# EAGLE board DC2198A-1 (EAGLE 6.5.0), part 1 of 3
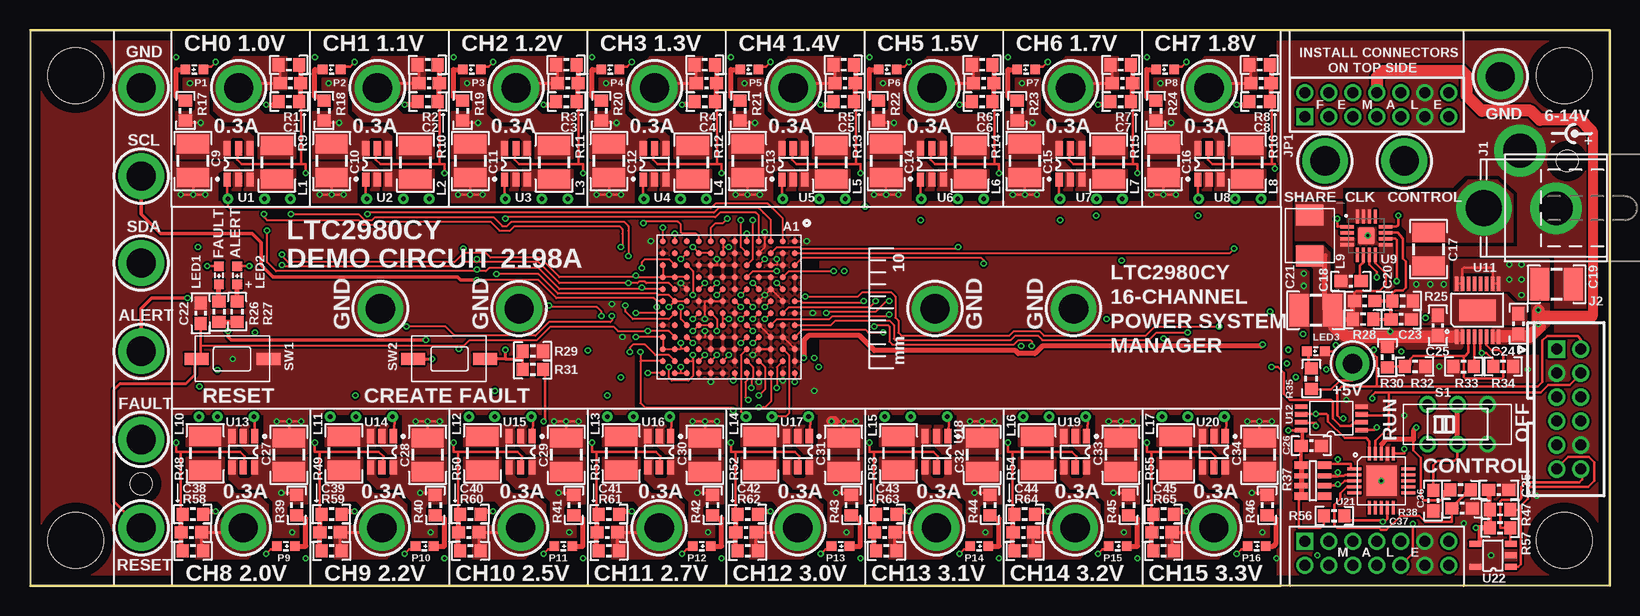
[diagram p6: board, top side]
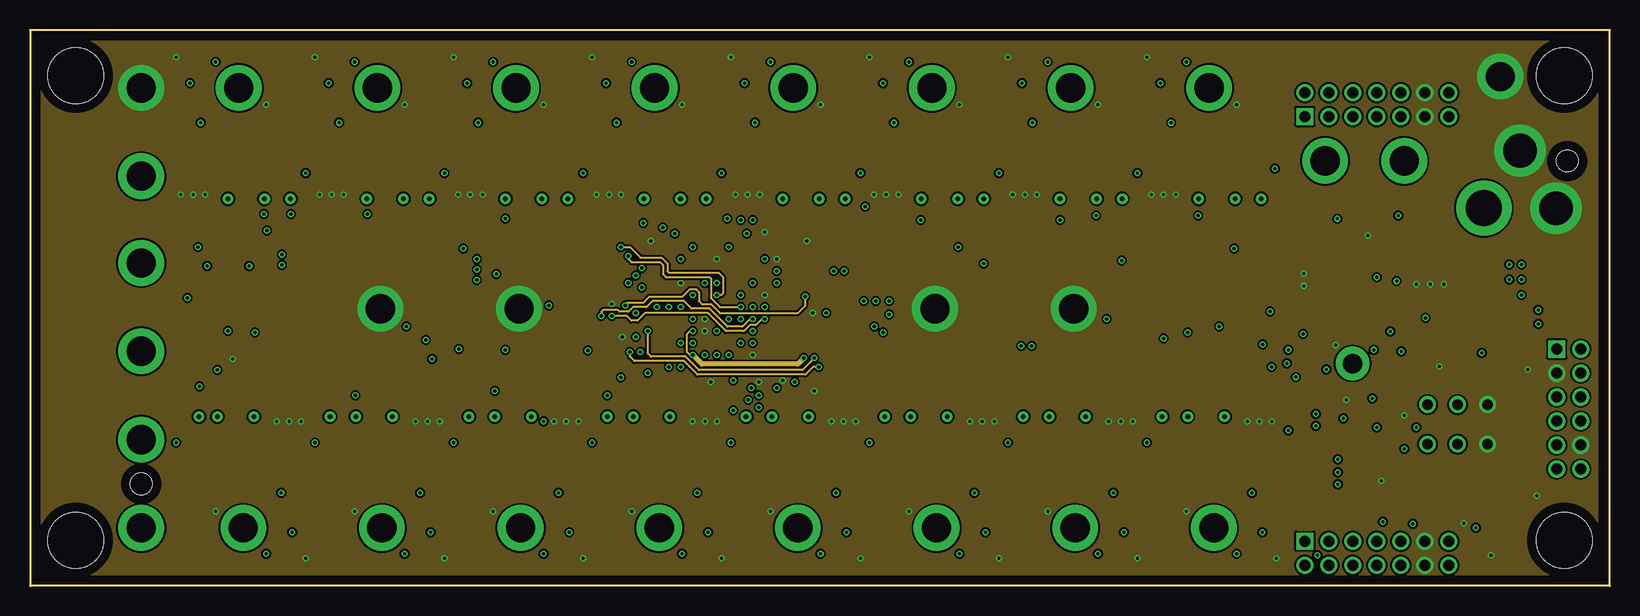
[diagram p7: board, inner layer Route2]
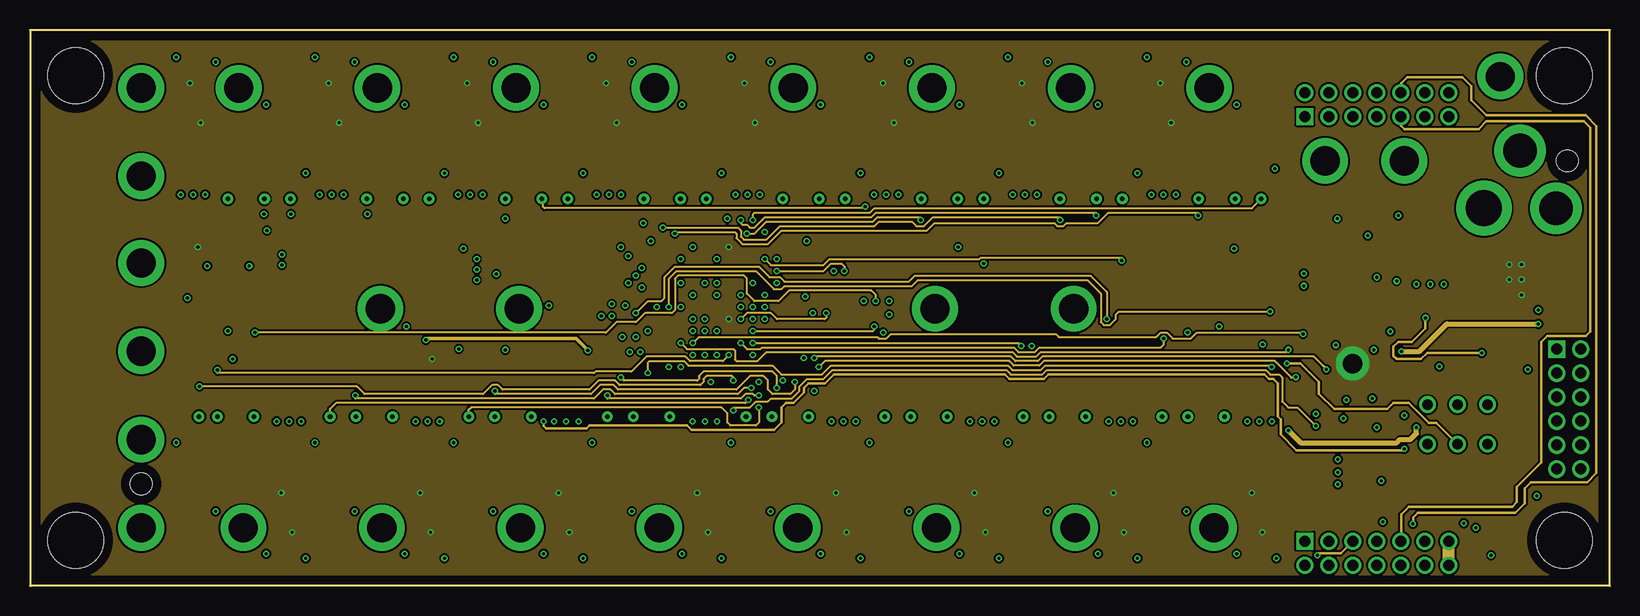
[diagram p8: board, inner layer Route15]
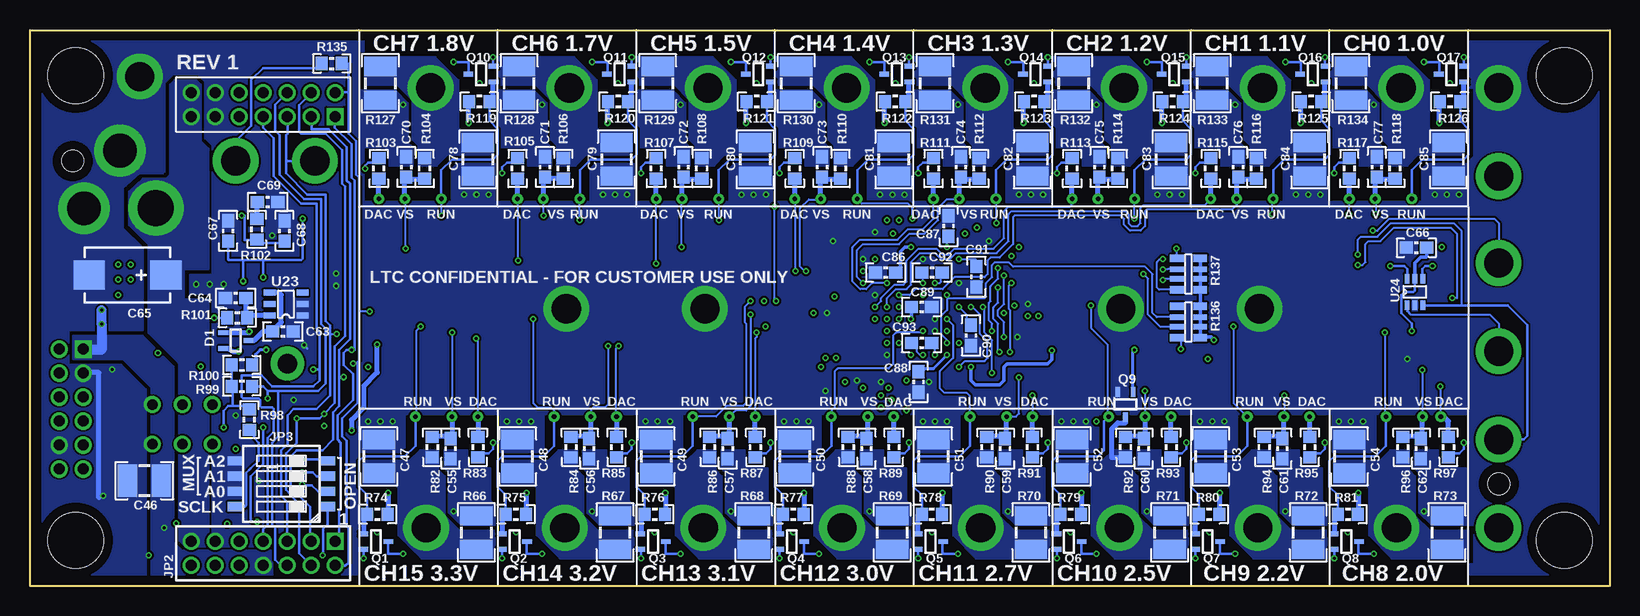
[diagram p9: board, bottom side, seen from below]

Size 131.7 x 46.35 mm. Coordinates in mm from the lower left corner, seen from the top.
Outline: 0,0 0,46.35 131.7,46.35 131.7,0 0.13,0
Copper layers (1*2+15*16): Top 0.035mm / dielectric 1.5mm / Route2 0.035mm / dielectric 0.15mm / Route15 0.035mm / dielectric 0.2mm / Bottom 0.035mm
Design rules "default *": minimum track width 6.5mil, minimum drill 10mil, track to track 0.16mm, track to pad 0.16mm, pad to pad 0.16mm, via to via 0.16mm, smd to smd 0.05mm, copper to edge 30mil, drill to drill 20mil, minimum pad ring 10mil, minimum via ring 5mil, stop-mask expansion 4mil, vias tented up to drill 16mil, thermal gap 10mil
Holes 4.65 mm at 3.81,3.81 3.81,42.55 127.89,42.55 127.89,3.81
Holes 1.8 mm at 9.27,8.51 128.14,35.43

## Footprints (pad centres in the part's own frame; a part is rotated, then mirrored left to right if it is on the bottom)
C0603_BOX = smd 1.1 x 1: 1 -0.85,0; 2 0.85,0
C1210_BOX = smd 1.6 x 2.7: 1 -1.4,0; 2 1.4,0
C7343 = smd 2.6 x 2.4: + -3.2,0; - 3.2,0
SC70-3 = smd 0.4 x 0.8: 1 -0.65,-1.052; 2 0.65,-1.052; 3 0,1.052
PJ-002A = drill 3 pad 4.6: 1 3,0 | drill 2.8 pad 4.3: 2 -3,0; 3 0,-4.8
CONN_DC1613 = drill 0.914 square: 1 -5,-1 | drill 0.914: 2 -5,1; 3 -3,-1; 4 -3,1; 5 -1,-1; 6 -1,1; 7 1,-1; 8 1,1; 9 3,-1; 10 3,1; 11 5,-1; 12 5,1
2X07M = drill 0.914 square: 1 -6,-1 | drill 0.914: 2 -6,1; 3 -4,-1; 4 -4,1; 5 -2,-1; 6 -2,1; 7 0,-1; 8 0,1; 9 2,-1; 10 2,1; 11 4,-1; 12 4,1; 13 6,-1; 14 6,1
SMT_DIP_4 = smd 1.27 x 0.762: 1 -3.861,1.905; 2 -3.861,0.635; 3 -3.861,-0.635; 4 -3.861,-1.905; 5 3.861,-1.905; 6 3.861,-0.635; 7 3.861,0.635; 8 3.861,1.905
L1210 = smd 1.6 x 2.7: 1 -1.4,0; 2 1.4,0
IHLP_1616AB = smd 1.75 x 2.3: 1 -1.7,0; 2 1.7,0
CHIPLED_0603 = smd 0.8 x 0.8: N 0,0.75; P 0,-0.75
R0603_BOX = smd 1 x 1.1: 1 -0.85,0; 2 0.85,0
R_VISHAY_CRA06S = smd 1.15 x 0.63: R1_1 -0.975,1.295; R1_2 0.975,1.295; R4_1 -0.975,-1.295; R4_2 0.975,-1.295 | smd 1.15 x 0.44: R2_1 -0.975,0.4; R2_2 0.975,0.4; R3_1 -0.975,-0.4; R3_2 0.975,-0.4
R1210_BOX = smd 1.6 x 2.7: 1 -1.4,0; 2 1.4,0
JS202011CQN = drill 0.9: 1 -2.5,1.65; 2 0,1.65; 3 2.5,1.65; 4 -2.5,-1.65; 5 0,-1.65; 6 2.5,-1.65
SWITCH_PTS635 = smd 2 x 1: SW1 -3,0; SW2 3,0
TP1 = drill 2.438 pad 3.81: TP 0,0
TURRET_SMALL_2308 = drill 1.626 pad 2.794: TP1 0,0
SOT-23-6 = smd 1.2 x 0.6: 1 -1.3,0.95; 2 -1.3,0; 3 -1.3,-0.95; 4 1.3,-0.95; 5 1.3,0; 6 1.3,0.95
QFN16_3X3 = smd 1.2 x 0.3: 1 -1.711,0.734; 2 -1.711,0.234; 3 -1.711,-0.266; 4 -1.711,-0.766; 9 1.489,-0.766; 10 1.489,-0.266; 11 1.489,0.234; 12 1.489,0.734 | smd 0.3 x 1.2: 5 -0.861,-1.616; 6 -0.361,-1.616; 7 0.139,-1.616; 8 0.639,-1.616; 13 0.639,1.584; 14 0.139,1.584; 15 -0.361,1.584; 16 -0.861,1.584 | smd 1.4 x 1.4: PAD -0.111,-0.016
BGA_144_1.0 = smd 0.5 x 0.5: A1 -5.5,5.5; A2 -4.5,5.5; A3 -3.5,5.5; A4 -2.5,5.5; A5 -1.5,5.5; A6 -0.5,5.5; A7 0.5,5.5; A8 1.5,5.5; A9 2.5,5.5; A10 3.5,5.5; A11 4.5,5.5; A12 5.5,5.5; B1 -5.5,4.5; B2 -4.5,4.5; B3 -3.5,4.5; B4 -2.5,4.5; B5 -1.5,4.5; B6 -0.5,4.5; B7 0.5,4.5; B8 1.5,4.5; B9 2.5,4.5; B10 3.5,4.5; B11 4.5,4.5; B12 5.5,4.5; C1 -5.5,3.5; C2 -4.5,3.5; C3 -3.5,3.5; C4 -2.5,3.5; C5 -1.5,3.5; C6 -0.5,3.5; C7 0.5,3.5; C8 1.5,3.5; C9 2.5,3.5; C10 3.5,3.5; C11 4.5,3.5; C12 5.5,3.5; D1 -5.5,2.5; D2 -4.5,2.5; D3 -3.5,2.5; D4 -2.5,2.5; D5 -1.5,2.5; D6 -0.5,2.5; D7 0.5,2.5; D8 1.5,2.5; D9 2.5,2.5; D10 3.5,2.5; D11 4.5,2.5; D12 5.5,2.5; E1 -5.5,1.5; E2 -4.5,1.5; E3 -3.5,1.5; E4 -2.5,1.5; E5 -1.5,1.5; E6 -0.5,1.5; E7 0.5,1.5; E8 1.5,1.5; E9 2.5,1.5; E10 3.5,1.5; E11 4.5,1.5; E12 5.5,1.5; F1 -5.5,0.5; F2 -4.5,0.5; F3 -3.5,0.5; F4 -2.5,0.5; F5 -1.5,0.5; F6 -0.5,0.5; F7 0.5,0.5; F8 1.5,0.5; F9 2.5,0.5; F10 3.5,0.5; F11 4.5,0.5; F12 5.5,0.5; G1 -5.5,-0.5; G2 -4.5,-0.5; G3 -3.5,-0.5; G4 -2.5,-0.5; G5 -1.5,-0.5; G6 -0.5,-0.5; G7 0.5,-0.5; G8 1.5,-0.5; G9 2.5,-0.5; G10 3.5,-0.5; G11 4.5,-0.5; G12 5.5,-0.5; H1 -5.5,-1.5; H2 -4.5,-1.5; H3 -3.5,-1.5; H4 -2.5,-1.5; H5 -1.5,-1.5; H6 -0.5,-1.5; H7 0.5,-1.5; H8 1.5,-1.5; H9 2.5,-1.5; H10 3.5,-1.5; H11 4.5,-1.5; H12 5.5,-1.5; J1 -5.5,-2.5; J2 -4.5,-2.5; J3 -3.5,-2.5; J4 -2.5,-2.5; J5 -1.5,-2.5; J6 -0.5,-2.5; J7 0.5,-2.5; J8 1.5,-2.5; J9 2.5,-2.5; J10 3.5,-2.5; J11 4.5,-2.5; J12 5.5,-2.5; K1 -5.5,-3.5; K2 -4.5,-3.5; K3 -3.5,-3.5; K4 -2.5,-3.5; K5 -1.5,-3.5; K6 -0.5,-3.5; K7 0.5,-3.5; K8 1.5,-3.5; K9 2.5,-3.5; K10 3.5,-3.5; K11 4.5,-3.5; K12 5.5,-3.5; L1 -5.5,-4.5; L2 -4.5,-4.5; L3 -3.5,-4.5; L4 -2.5,-4.5; L5 -1.5,-4.5; L6 -0.5,-4.5; L7 0.5,-4.5; L8 1.5,-4.5; L9 2.5,-4.5; L10 3.5,-4.5; L11 4.5,-4.5; L12 5.5,-4.5; M1 -5.5,-5.5; M2 -4.5,-5.5; M3 -3.5,-5.5; M4 -2.5,-5.5; M5 -1.5,-5.5; M6 -0.5,-5.5; M7 0.5,-5.5; M8 1.5,-5.5; M9 2.5,-5.5; M10 3.5,-5.5; M11 4.5,-5.5; M12 5.5,-5.5
MSOP16_EXP = smd 1.2 x 0.3: 1 -2.213,1.75; 2 -2.213,1.25; 3 -2.213,0.75; 4 -2.213,0.25; 5 -2.213,-0.25; 6 -2.213,-0.75; 7 -2.213,-1.25; 8 -2.213,-1.75; 9 2.213,-1.75; 10 2.213,-1.25; 11 2.213,-0.75; 12 2.213,-0.25; 13 2.213,0.25; 14 2.213,0.75; 15 2.213,1.25; 16 2.213,1.75 | smd 1.778 x 3.048: EXP 0,0
MSOP-8 = smd 1.041 x 0.381: 1 -2.55,0.975; 2 -2.55,0.325; 3 -2.55,-0.325; 4 -2.55,-0.975; 5 2.479,-0.975; 6 2.479,-0.325; 7 2.479,0.325; 8 2.479,0.975
QFN20 = smd 1.143 x 0.254: 1 -2.25,1; 2 -2.25,0.5; 3 -2.25,0; 4 -2.25,-0.5; 5 -2.25,-1; 11 2.25,-1; 12 2.25,-0.5; 13 2.25,0; 14 2.25,0.5; 15 2.25,1 | smd 0.254 x 1.143: 6 -1,-2.25; 7 -0.5,-2.25; 8 0,-2.25; 9 0.5,-2.25; 10 1,-2.25; 16 1,2.25; 17 0.5,2.25; 18 0,2.25; 19 -0.5,2.25; 20 -1,2.25 | smd 2.54 x 2.54: PAD 0,0
SOT-23-5 = smd 1 x 0.5: 1 -1.649,0.95; 2 -1.649,0; 3 -1.649,-0.95; 4 1.333,-0.95; 5 1.333,0.95
SOT-23-6@1 = smd 1 x 0.5: 1 -1.374,1.087; 2 -1.374,0.127; 3 -1.374,-0.833; 4 1.374,-0.833; 5 1.374,0.127; 6 1.374,1.087
SC70-6 = smd 0.4 x 0.8: 1 -0.65,-1.102; 2 0,-1.102; 3 0.65,-1.102; 4 0.65,1.102; 5 0,1.098; 6 -0.65,1.102
VIA = drill 0.381: 1 0,0

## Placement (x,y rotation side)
$$U$1  [LT_LOGO_LARGE_SM]  5.46,6.1 90 top
$$U$2  [LT_LOGO_LARGE_SM]  2.03,6.1 90 bottom
C1  220p  [C0603_BOX]  21.72,41.91 0 top
C2  220p  [C0603_BOX]  33.27,41.91 0 top
C3  220p  [C0603_BOX]  44.83,41.91 0 top
C4  220p  [C0603_BOX]  56.39,41.91 0 top
C5  220p  [C0603_BOX]  67.94,41.91 0 top
C6  220p  [C0603_BOX]  79.5,41.91 0 top
C7  220p  [C0603_BOX]  91.06,41.91 0 top
C8  220p  [C0603_BOX]  102.62,41.91 0 top
C9  10u/10V  [C1210_BOX]  13.59,35.43 270 top
C10  10u/10V  [C1210_BOX]  25.15,35.43 270 top
C11  10u/10V  [C1210_BOX]  36.7,35.43 270 top
C12  10u/10V  [C1210_BOX]  48.26,35.43 270 top
C13  10u/10V  [C1210_BOX]  59.82,35.43 270 top
C14  10u/10V  [C1210_BOX]  71.37,35.43 270 top
C15  10u/10V  [C1210_BOX]  82.93,35.43 270 top
C16  10u/10V  [C1210_BOX]  94.49,35.43 270 top
C17  10u/25V  [C1210_BOX]  116.59,28.07 90 top
C18  100n  [C0603_BOX]  110.11,25.4 0 top
C19  10u/10V  [C1210_BOX]  127.25,25.15 0 top
C20  68p  [C0603_BOX]  111.25,23.75 0 top
C21  22u/10V  [C1210_BOX]  107.19,22.99 180 top
C22  10n  [C0603_BOX]  14.22,22.73 90 top
C23  47p  [C0603_BOX]  114.3,22.23 0 top
C24  1u  [C0603_BOX]  124.08,21.84 90 top
C25  1u  [C0603_BOX]  117.35,21.72 90 top
C26  100n  [C0603_BOX]  106.81,11.68 0 top
C27  10u/10V  [C1210_BOX]  21.59,10.92 90 top
C28  10u/10V  [C1210_BOX]  33.15,10.92 90 top
C29  10u/10V  [C1210_BOX]  44.7,10.92 90 top
C30  10u/10V  [C1210_BOX]  56.26,10.92 90 top
C31  10u/10V  [C1210_BOX]  67.82,10.92 90 top
C32  10u/10V  [C1210_BOX]  79.38,10.92 90 top
C33  10u/10V  [C1210_BOX]  90.93,10.92 90 top
C34  10u/10V  [C1210_BOX]  102.49,10.92 90 top
C35  1u  [C0603_BOX]  122.43,8 0 top
C36  1u  [C0603_BOX]  116.97,7.11 270 top
C37  1u  [C0603_BOX]  119.38,6.48 0 top
C38  220p  [C0603_BOX]  13.46,4.45 180 top
C39  220p  [C0603_BOX]  25.02,4.45 180 top
C40  220p  [C0603_BOX]  36.58,4.45 180 top
C41  220p  [C0603_BOX]  48.13,4.45 180 top
C42  220p  [C0603_BOX]  59.69,4.45 180 top
C43  220p  [C0603_BOX]  71.25,4.45 180 top
C44  220p  [C0603_BOX]  82.8,4.45 180 top
C45  220p  [C0603_BOX]  94.36,4.45 180 top
C46  10u/10V  [C1210_BOX]  122.17,8.76 180 bottom
C47  22u/10V  [C1210_BOX]  102.62,10.79 90 bottom
C48  22u/10V  [C1210_BOX]  91.06,10.79 90 bottom
C49  22u/10V  [C1210_BOX]  79.5,10.79 90 bottom
C50  22u/10V  [C1210_BOX]  67.94,10.79 90 bottom
C51  22u/10V  [C1210_BOX]  56.39,10.79 90 bottom
C52  22u/10V  [C1210_BOX]  44.83,10.79 90 bottom
C53  22u/10V  [C1210_BOX]  33.27,10.79 90 bottom
C54  22u/10V  [C1210_BOX]  21.72,10.79 90 bottom
C55  100n  [C0603_BOX]  96.65,11.43 90 bottom
C56  100n  [C0603_BOX]  85.09,11.43 90 bottom
C57  100n  [C0603_BOX]  73.53,11.43 90 bottom
C58  100n  [C0603_BOX]  61.98,11.43 90 bottom
C59  100n  [C0603_BOX]  50.42,11.43 90 bottom
C60  100n  [C0603_BOX]  38.86,11.43 90 bottom
C61  100n  [C0603_BOX]  27.3,11.43 90 bottom
C62  100n  [C0603_BOX]  15.75,11.43 90 bottom
C63  1u  [C0603_BOX]  110.62,21.21 0 bottom
C64  4.7u  [C0603_BOX]  114.55,24 0 bottom
C65  47u/16V  [C7343]  123.57,25.91 180 bottom
C66  1u  [C0603_BOX]  16.13,28.19 180 bottom
C67  4.7u  [C0603_BOX]  115.19,29.59 90 bottom
C68  4.7p  [C0603_BOX]  110.49,29.59 90 bottom
C69  68p  [C0603_BOX]  111.89,32 0 bottom
C70  100n  [C0603_BOX]  100.33,34.92 270 bottom
C71  100n  [C0603_BOX]  88.77,34.92 270 bottom
C72  100n  [C0603_BOX]  77.22,34.92 270 bottom
C73  100n  [C0603_BOX]  65.66,34.92 270 bottom
C74  100n  [C0603_BOX]  54.1,34.92 270 bottom
C75  100n  [C0603_BOX]  42.55,34.92 270 bottom
C76  100n  [C0603_BOX]  30.99,34.92 270 bottom
C77  100n  [C0603_BOX]  19.43,34.92 270 bottom
C78  22u/10V  [C1210_BOX]  94.36,35.56 270 bottom
C79  22u/10V  [C1210_BOX]  82.8,35.56 270 bottom
C80  22u/10V  [C1210_BOX]  71.25,35.56 270 bottom
C81  22u/10V  [C1210_BOX]  59.69,35.56 270 bottom
C82  22u/10V  [C1210_BOX]  48.13,35.56 270 bottom
C83  22u/10V  [C1210_BOX]  36.58,35.56 270 bottom
C84  22u/10V  [C1210_BOX]  25.02,35.56 270 bottom
C85  22u/10V  [C1210_BOX]  13.46,35.56 270 bottom
C86  100n  [C0603_BOX]  60.38,26.12 180 bottom
C87  100n  [C0603_BOX]  55.12,30 90 bottom
C88  100n  [C0603_BOX]  57.62,17 90 bottom
C89  100n  [C0603_BOX]  57.38,23.25 0 bottom
C90  100n  [C0603_BOX]  53.25,20.88 90 bottom
C91  100n  [C0603_BOX]  52.81,25.78 90 bottom
C92  100n  [C0603_BOX]  56.5,26.12 180 bottom
C93  100n  [C0603_BOX]  57.38,20.25 180 bottom
D1  BAT30CWFILM  [SC70-3]  114.55,20.45 270 bottom
DRILEGEND  [DRILEGEND]  not placed on the board
J1  PJ-002A  [PJ-002A]  124.21,31.5 180 top
J2  CONN_DC1613  [CONN_DC1613]  128.27,14.73 270 top
JP1  FEMALE  [2X07M]  112.27,40.13 0 top
JP2  MALE  [2X07M]  112.27,2.72 180 bottom
JP3  TDA04H0SK1  [SMT_DIP_4]  110.74,8.51 0 bottom
L1  4.7uH  [L1210]  20.57,35.31 90 top
L2  4.7uH  [L1210]  32.13,35.31 90 top
L3  4.7uH  [L1210]  43.69,35.31 90 top
L4  4.7uH  [L1210]  55.24,35.31 90 top
L5  4.7uH  [L1210]  66.8,35.31 90 top
L6  4.7uH  [L1210]  78.36,35.31 90 top
L7  4.7uH  [L1210]  89.92,35.31 90 top
L8  4.7uH  [L1210]  101.47,35.31 90 top
L9  2.2uH  [IHLP_1616AB]  106.68,29.21 270 top
L10  4.7uH  [L1210]  14.61,11.05 270 top
L11  4.7uH  [L1210]  26.16,11.05 270 top
L12  4.7uH  [L1210]  37.72,11.05 270 top
L13  4.7uH  [L1210]  49.28,11.05 270 top
L14  4.7uH  [L1210]  60.83,11.05 270 top
L15  4.7uH  [L1210]  72.39,11.05 270 top
L16  4.7uH  [L1210]  83.95,11.05 270 top
L17  4.7uH  [L1210]  95.5,11.05 270 top
LED1  RED  [CHIPLED_0603]  15.75,25.91 0 top
LED2  RED  [CHIPLED_0603]  17.27,25.91 0 top
LED3  GREEN  [CHIPLED_0603]  107.19,19.56 270 top
P1  GREEN  [CHIPLED_0603]  13.72,43.05 270 top
P2  GREEN  [CHIPLED_0603]  25.15,43.05 270 top
P3  GREEN  [CHIPLED_0603]  36.83,43.05 270 top
P4  GREEN  [CHIPLED_0603]  48.39,43.05 270 top
P5  GREEN  [CHIPLED_0603]  59.94,43.05 270 top
P6  GREEN  [CHIPLED_0603]  71.5,43.05 270 top
P7  GREEN  [CHIPLED_0603]  83.06,43.05 270 top
P8  GREEN  [CHIPLED_0603]  94.61,43.05 270 top
P9  GREEN  [CHIPLED_0603]  21.34,3.3 90 top
P10  GREEN  [CHIPLED_0603]  32.89,3.3 90 top
P11  GREEN  [CHIPLED_0603]  44.45,3.3 90 top
P12  GREEN  [CHIPLED_0603]  56.01,3.3 90 top
P13  GREEN  [CHIPLED_0603]  67.56,3.3 90 top
P14  GREEN  [CHIPLED_0603]  79.12,3.3 90 top
P15  GREEN  [CHIPLED_0603]  90.68,3.3 90 top
P16  GREEN  [CHIPLED_0603]  102.23,3.3 90 top
Q1  Si1308EDL  [SC70-3]  102.87,3.68 270 bottom
Q2  Si1308EDL  [SC70-3]  91.31,3.68 270 bottom
Q3  Si1308EDL  [SC70-3]  79.76,3.68 270 bottom
Q4  Si1308EDL  [SC70-3]  68.2,3.68 270 bottom
Q5  Si1308EDL  [SC70-3]  56.64,3.68 270 bottom
Q6  Si1308EDL  [SC70-3]  45.09,3.68 270 bottom
Q7  Si1308EDL  [SC70-3]  33.53,3.68 270 bottom
Q8  Si1308EDL  [SC70-3]  21.97,3.68 270 bottom
Q9  Si1308EDL  [SC70-3]  40.39,15.11 180 bottom
Q10  Si1308EDL  [SC70-3]  94.11,42.67 90 bottom
Q11  Si1308EDL  [SC70-3]  82.55,42.67 90 bottom
Q12  Si1308EDL  [SC70-3]  70.99,42.67 90 bottom
Q13  Si1308EDL  [SC70-3]  59.44,42.67 90 bottom
Q14  Si1308EDL  [SC70-3]  47.88,42.67 90 bottom
Q15  Si1308EDL  [SC70-3]  36.32,42.67 90 bottom
Q16  Si1308EDL  [SC70-3]  24.77,42.67 90 bottom
Q17  Si1308EDL  [SC70-3]  13.21,42.67 90 bottom
R1  100k  [R0603_BOX]  21.59,43.43 180 top
R2  100k  [R0603_BOX]  33.15,43.43 180 top
R3  100k  [R0603_BOX]  44.7,43.43 180 top
R4  100k  [R0603_BOX]  56.26,43.43 180 top
R5  100k  [R0603_BOX]  67.82,43.43 180 top
R6  100k  [R0603_BOX]  79.38,43.43 180 top
R7  100k  [R0603_BOX]  90.93,43.43 180 top
R8  100k  [R0603_BOX]  102.49,43.43 180 top
R9  402k  [R0603_BOX]  21.59,40.39 0 top
R10  267k  [R0603_BOX]  33.15,40.39 0 top
R11  200k  [R0603_BOX]  44.7,40.39 0 top
R12  158k  [R0603_BOX]  56.26,40.39 0 top
R13  133k  [R0603_BOX]  67.82,40.39 0 top
R14  115k  [R0603_BOX]  79.38,40.39 0 top
R15  88.7k  [R0603_BOX]  90.93,40.39 0 top
R16  80.6k  [R0603_BOX]  102.49,40.39 0 top
R17  3.01k  [R0603_BOX]  12.95,39.62 270 top
R18  3.01k  [R0603_BOX]  24.51,39.62 270 top
R19  3.01k  [R0603_BOX]  36.07,39.62 270 top
R20  3.01k  [R0603_BOX]  47.62,39.62 270 top
R21  3.01k  [R0603_BOX]  59.18,39.62 270 top
R22  3.01k  [R0603_BOX]  70.74,39.62 270 top
R23  3.01k  [R0603_BOX]  82.3,39.62 270 top
R24  3.01k  [R0603_BOX]  93.85,39.62 270 top
R25  10k  [R0603_BOX]  114.43,23.75 180 top
R26  698  [R0603_BOX]  15.75,22.86 90 top
R27  698  [R0603_BOX]  17.27,22.86 270 top
R28  73.2k  [R0603_BOX]  111.12,22.23 180 top
R29  100k  [R0603_BOX]  41.91,19.56 180 top
R30  46.4k  [R0603_BOX]  113.16,19.05 90 top
R31  OPT  [R0603_BOX]  41.91,18.04 180 top
R32  10k  [R0603_BOX]  115.44,18.29 180 top
R33  249  [R0603_BOX]  119.51,18.29 0 top
R34  1.0k  [R0603_BOX]  122.81,18.29 180 top
R35  3.01k  [R0603_BOX]  106.81,17.27 270 top
R37  10k, 4X  [R_VISHAY_CRA06S]  106.93,8.76 180 top
R38  249  [R0603_BOX]  119.25,8 0 top
R39  3.01k  [R0603_BOX]  22.23,6.73 90 top
R40  3.01k  [R0603_BOX]  33.78,6.73 90 top
R41  3.01k  [R0603_BOX]  45.34,6.73 90 top
R42  3.01k  [R0603_BOX]  56.9,6.73 90 top
R43  3.01k  [R0603_BOX]  68.45,6.73 90 top
R44  3.01k  [R0603_BOX]  80.01,6.73 90 top
R45  3.01k  [R0603_BOX]  91.57,6.73 90 top
R46  3.01k  [R0603_BOX]  103.12,6.73 90 top
R47  10k  [R0603_BOX]  122.56,6.35 180 top
R48  66.5k  [R0603_BOX]  13.59,5.97 180 top
R49  57.6k  [R0603_BOX]  25.15,5.97 180 top
R50  47.5k  [R0603_BOX]  36.7,5.97 180 top
R51  42.2k  [R0603_BOX]  48.26,5.97 180 top
R52  36.5k  [R0603_BOX]  59.82,5.97 180 top
R53  34.8k  [R0603_BOX]  71.37,5.97 180 top
R54  33.2k  [R0603_BOX]  82.93,5.97 180 top
R55  32.4k  [R0603_BOX]  94.49,5.97 180 top
R56  10k  [R0603_BOX]  108.71,5.84 0 top
R57  10k  [R0603_BOX]  122.56,4.83 180 top
R58  100k  [R0603_BOX]  13.59,2.92 0 top
R59  100k  [R0603_BOX]  25.15,2.92 0 top
R60  100k  [R0603_BOX]  36.7,2.92 0 top
R61  100k  [R0603_BOX]  48.26,2.92 0 top
R62  100k  [R0603_BOX]  59.82,2.92 0 top
R63  100k  [R0603_BOX]  71.37,2.92 0 top
R64  100k  [R0603_BOX]  82.93,2.92 0 top
R65  100k  [R0603_BOX]  94.49,2.92 0 top
R66  470  [R1210_BOX]  94.49,4.45 270 bottom
R67  470  [R1210_BOX]  82.93,4.45 270 bottom
R68  470  [R1210_BOX]  71.37,4.45 270 bottom
R69  470  [R1210_BOX]  59.82,4.45 270 bottom
R70  470  [R1210_BOX]  48.26,4.45 270 bottom
R71  470  [R1210_BOX]  36.7,4.45 270 bottom
R72  470  [R1210_BOX]  25.15,4.45 270 bottom
R73  470  [R1210_BOX]  13.59,4.45 270 bottom
R74  100k  [R0603_BOX]  102.74,5.97 0 bottom
R75  100k  [R0603_BOX]  91.19,5.97 0 bottom
R76  100k  [R0603_BOX]  79.63,5.97 0 bottom
R77  100k  [R0603_BOX]  68.07,5.97 0 bottom
R78  100k  [R0603_BOX]  56.52,5.97 0 bottom
R79  100k  [R0603_BOX]  44.96,5.97 0 bottom
R80  100k  [R0603_BOX]  33.4,5.97 0 bottom
R81  100k  [R0603_BOX]  21.84,5.97 0 bottom
R82  100  [R0603_BOX]  98.17,11.56 90 bottom
R83  182k  [R0603_BOX]  94.36,11.56 90 bottom
R84  100  [R0603_BOX]  86.61,11.56 90 bottom
R85  191k  [R0603_BOX]  82.8,11.56 90 bottom
R86  100  [R0603_BOX]  75.06,11.56 90 bottom
R87  196k  [R0603_BOX]  71.25,11.56 90 bottom
R88  100  [R0603_BOX]  63.5,11.56 90 bottom
R89  205k  [R0603_BOX]  59.69,11.56 90 bottom
R90  100  [R0603_BOX]  51.94,11.56 90 bottom
R91  226k  [R0603_BOX]  48.13,11.56 90 bottom
R92  100  [R0603_BOX]  40.39,11.56 90 bottom
R93  243k  [R0603_BOX]  36.58,11.56 90 bottom
R94  100  [R0603_BOX]  28.83,11.56 90 bottom
R95  274k  [R0603_BOX]  25.02,11.56 90 bottom
R96  100  [R0603_BOX]  17.27,11.56 90 bottom
R97  301k  [R0603_BOX]  13.46,11.56 90 bottom
R98  10k  [R0603_BOX]  113.41,13.84 270 bottom
R99  10k  [R0603_BOX]  114.05,16.64 0 bottom
R100  10k  [R0603_BOX]  114.05,18.41 0 bottom
R101  2.49k  [R0603_BOX]  114.43,22.35 0 bottom
R102  73.2k  [R0603_BOX]  112.78,29.72 270 bottom
R103  340k  [R0603_BOX]  102.62,34.8 270 bottom
R104  100  [R0603_BOX]  98.81,34.8 270 bottom
R105  357k  [R0603_BOX]  91.06,34.8 270 bottom
R106  100  [R0603_BOX]  87.25,34.8 270 bottom
R107  402k  [R0603_BOX]  79.5,34.8 270 bottom
R108  100  [R0603_BOX]  75.69,34.8 270 bottom
R109  374k  [R0603_BOX]  67.94,34.8 270 bottom
R110  100  [R0603_BOX]  64.14,34.8 270 bottom
R111  464k  [R0603_BOX]  56.39,34.8 270 bottom
R112  100  [R0603_BOX]  52.58,34.8 270 bottom
R113  511k  [R0603_BOX]  44.83,34.8 270 bottom
R114  100  [R0603_BOX]  41.02,34.8 270 bottom
R115  549k  [R0603_BOX]  33.27,34.8 270 bottom
R116  100  [R0603_BOX]  29.46,34.8 270 bottom
R117  604k  [R0603_BOX]  21.72,34.8 270 bottom
R118  100  [R0603_BOX]  17.91,34.8 270 bottom
R119  100k  [R0603_BOX]  94.23,40.39 180 bottom
R120  100k  [R0603_BOX]  82.68,40.39 180 bottom
R121  100k  [R0603_BOX]  71.12,40.39 180 bottom
R122  100k  [R0603_BOX]  59.56,40.39 180 bottom
R123  100k  [R0603_BOX]  48.01,40.39 180 bottom
R124  100k  [R0603_BOX]  36.45,40.39 180 bottom
R125  100k  [R0603_BOX]  24.89,40.39 180 bottom
R126  100k  [R0603_BOX]  13.34,40.39 180 bottom
R127  470  [R1210_BOX]  102.49,41.91 90 bottom
R128  470  [R1210_BOX]  90.93,41.91 90 bottom
R129  470  [R1210_BOX]  79.38,41.91 90 bottom
R130  470  [R1210_BOX]  67.82,41.91 90 bottom
R131  470  [R1210_BOX]  56.26,41.91 90 bottom
R132  470  [R1210_BOX]  44.7,41.91 90 bottom
R133  470  [R1210_BOX]  33.15,41.91 90 bottom
R134  470  [R1210_BOX]  21.59,41.91 90 bottom
R135  10k  [R0603_BOX]  106.55,43.56 0 bottom
R136  10k, 4X  [R_VISHAY_CRA06S]  35.12,22 180 bottom
R137  10k, 4X  [R_VISHAY_CRA06S]  35.12,26 0 bottom
S1  CONTROL  [JS202011CQN]  119,13.46 0 top
SW1  PTS635SL25SMTR LFS  [SWITCH_PTS635]  16.89,18.92 0 top
SW2  PTS635SK25SMTR LFS  [SWITCH_PTS635]  34.92,18.92 180 top
TP1  TESTPOINT_BIG  [TP1]  122.56,42.47 0 top
TP2  TESTPOINT_BIG  [TP1]  9.27,41.53 0 top
TP3  TESTPOINT_BIG  [TP1]  17.4,41.53 90 top
TP4  TESTPOINT_BIG  [TP1]  28.96,41.53 90 top
TP5  TESTPOINT_BIG  [TP1]  40.51,41.53 90 top
TP6  TESTPOINT_BIG  [TP1]  52.07,41.53 90 top
TP7  TESTPOINT_BIG  [TP1]  63.63,41.53 90 top
TP8  TESTPOINT_BIG  [TP1]  75.18,41.53 90 top
TP9  TESTPOINT_BIG  [TP1]  86.74,41.53 90 top
TP10  TESTPOINT_BIG  [TP1]  98.3,41.53 90 top
TP11  TESTPOINT_BIG  [TP1]  107.95,35.43 0 top
TP12  TESTPOINT_BIG  [TP1]  114.55,35.43 0 top
TP13  TESTPOINT_BIG  [TP1]  9.27,34.16 0 top
TP14  TESTPOINT_BIG  [TP1]  9.27,26.92 0 top
TP15  TESTPOINT_BIG  [TP1]  29.21,23.11 0 top
TP16  TESTPOINT_BIG  [TP1]  40.77,23.11 0 top
TP17  TESTPOINT_BIG  [TP1]  75.44,23.11 0 top
TP18  TESTPOINT_BIG  [TP1]  87,23.11 0 top
TP19  TESTPOINT_BIG  [TP1]  9.27,19.56 0 top
TP20  TURRET_SMALL_2308TP  [TURRET_SMALL_2308]  110.24,18.54 0 top
TP21  TESTPOINT_BIG  [TP1]  9.27,12.19 0 top
TP22  TESTPOINT_BIG  [TP1]  9.27,4.83 0 top
TP23  TESTPOINT_BIG  [TP1]  17.78,4.83 270 top
TP24  TESTPOINT_BIG  [TP1]  29.34,4.83 270 top
TP25  TESTPOINT_BIG  [TP1]  40.89,4.83 270 top
TP26  TESTPOINT_BIG  [TP1]  52.45,4.83 270 top
TP27  TESTPOINT_BIG  [TP1]  64.01,4.83 270 top
TP28  TESTPOINT_BIG  [TP1]  75.56,4.83 270 top
TP29  TESTPOINT_BIG  [TP1]  87.12,4.83 270 top
TP30  TESTPOINT_BIG  [TP1]  98.68,4.83 270 top
U1  LTC3405AES6  [SOT-23-6]  17.4,35.18 90 top
U2  LTC3405AES6  [SOT-23-6]  28.96,35.18 90 top
U3  LTC3405AES6  [SOT-23-6]  40.51,35.18 90 top
U4  LTC3405AES6  [SOT-23-6]  52.07,35.18 90 top
U5  LTC3405AES6  [SOT-23-6]  63.63,35.18 90 top
U6  LTC3405AES6  [SOT-23-6]  75.18,35.18 90 top
U7  LTC3405AES6  [SOT-23-6]  86.74,35.18 90 top
U8  LTC3405AES6  [SOT-23-6]  98.3,35.18 90 top
U9  LTC3604IUD  [QFN16_3X3]  111.51,29.21 0 top
U10  LTC2980CY  [BGA_144_1.0]  58.25,23.25 270 top
U11  LTC4415IMSE  [MSOP16_EXP]  120.65,22.99 90 top
U12  LTC4313CMS8  [MSOP-8]  108.46,13.97 180 top
U13  LTC3405AES6  [SOT-23-6]  17.78,11.18 270 top
U14  LTC3405AES6  [SOT-23-6]  29.34,11.18 270 top
U15  LTC3405AES6  [SOT-23-6]  40.89,11.18 270 top
U16  LTC3405AES6  [SOT-23-6]  52.45,11.18 270 top
U17  LTC3405AES6  [SOT-23-6]  64.01,11.18 270 top
U18  LTC3405AES6  [SOT-23-6]  75.56,11.18 270 top
U19  LTC3405AES6  [SOT-23-6]  87.12,11.18 270 top
U20  LTC3405AES6  [SOT-23-6]  98.68,11.18 270 top
U21  MCP23008-E/ML  [QFN20]  112.65,8.76 0 top
U22  24AA02T-I/OT  [SOT-23-5]  121.79,2.54 180 top
U23  LT6654BMPS6-1.25  [SOT-23-6@1]  110.36,23.62 180 bottom
U24  SN74LVC2G34DCK  [SC70-6]  16.26,24.51 0 bottom
U$49  [RULER]  69.98,18.16 90 top
U$73  [DC2198_FRAME]  not placed on the board
VSNSN1  TESPOINT_SMD  [VIA]  16.51,32.26 180 top
VSNSN2  TESPOINT_SMD  [VIA]  28.07,32.26 180 top
VSNSN3  TESPOINT_SMD  [VIA]  39.62,32.26 180 top
VSNSN4  TESPOINT_SMD  [VIA]  51.18,32.26 180 top
VSNSN5  TESPOINT_SMD  [VIA]  62.74,32.26 180 top
VSNSN6  TESPOINT_SMD  [VIA]  74.3,32.26 180 top
VSNSN7  TESPOINT_SMD  [VIA]  85.85,32.26 180 top
VSNSN8  TESPOINT_SMD  [VIA]  97.41,32.26 180 top
VSNSN9  TESPOINT_SMD  [VIA]  18.67,14.1 0 top
VSNSN10  TESPOINT_SMD  [VIA]  30.23,14.1 0 top
VSNSN11  TESPOINT_SMD  [VIA]  41.78,14.1 0 top
VSNSN12  TESPOINT_SMD  [VIA]  53.34,14.1 0 top
VSNSN13  TESPOINT_SMD  [VIA]  64.9,14.1 0 top
VSNSN14  TESPOINT_SMD  [VIA]  76.45,14.1 0 top
VSNSN15  TESPOINT_SMD  [VIA]  88.01,14.1 0 top
VSNSN16  TESPOINT_SMD  [VIA]  99.57,14.1 0 top
VSNSN17  TESPOINT_SMD  [VIA]  96.52,14.1 0 bottom
VSNSN18  TESPOINT_SMD  [VIA]  94.36,14.1 0 bottom
VSNSN19  TESPOINT_SMD  [VIA]  84.96,14.1 0 bottom
VSNSN20  TESPOINT_SMD  [VIA]  82.8,14.1 0 bottom
VSNSN21  TESPOINT_SMD  [VIA]  73.41,14.1 0 bottom
VSNSN22  TESPOINT_SMD  [VIA]  71.25,14.1 0 bottom
VSNSN23  TESPOINT_SMD  [VIA]  61.85,14.1 0 bottom
VSNSN24  TESPOINT_SMD  [VIA]  59.69,14.1 0 bottom
VSNSN25  TESPOINT_SMD  [VIA]  50.29,14.1 0 bottom
VSNSN26  TESPOINT_SMD  [VIA]  48.13,14.1 0 bottom
VSNSN27  TESPOINT_SMD  [VIA]  38.73,14.1 0 bottom
VSNSN28  TESPOINT_SMD  [VIA]  36.58,14.1 0 bottom
VSNSN29  TESPOINT_SMD  [VIA]  27.18,14.1 0 bottom
VSNSN30  TESPOINT_SMD  [VIA]  25.02,14.1 0 bottom
VSNSN31  TESPOINT_SMD  [VIA]  15.62,14.1 0 bottom
VSNSN32  TESPOINT_SMD  [VIA]  14.1,14.1 0 bottom
VSNSN33  TESPOINT_SMD  [VIA]  102.62,32.26 180 bottom
VSNSN34  TESPOINT_SMD  [VIA]  100.46,32.26 180 bottom
VSNSN35  TESPOINT_SMD  [VIA]  91.06,32.26 180 bottom
VSNSN36  TESPOINT_SMD  [VIA]  88.9,32.26 180 bottom
VSNSN37  TESPOINT_SMD  [VIA]  79.5,32.26 180 bottom
VSNSN38  TESPOINT_SMD  [VIA]  77.34,32.26 180 bottom
VSNSN39  TESPOINT_SMD  [VIA]  67.94,32.26 180 bottom
VSNSN40  TESPOINT_SMD  [VIA]  65.79,32.26 180 bottom
VSNSN41  TESPOINT_SMD  [VIA]  56.39,32.26 180 bottom
VSNSN42  TESPOINT_SMD  [VIA]  54.23,32.26 180 bottom
VSNSN43  TESPOINT_SMD  [VIA]  44.83,32.26 180 bottom
VSNSN44  TESPOINT_SMD  [VIA]  42.67,32.26 180 bottom
VSNSN45  TESPOINT_SMD  [VIA]  33.27,32.26 180 bottom
VSNSN46  TESPOINT_SMD  [VIA]  31.11,32.26 180 bottom
VSNSN47  TESPOINT_SMD  [VIA]  21.72,32.26 180 bottom
VSNSN48  TESPOINT_SMD  [VIA]  19.56,32.26 180 bottom

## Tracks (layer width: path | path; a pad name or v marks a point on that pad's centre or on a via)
+3V3  (via drill 0.25)
  Top 0.165: U10.H8 U10.J8 v55.25,21.25 | U10.K11 55.25,18.75 v55.25,19.25 55.25,17.5 54.88,17.12 53.5,17.12 53.25,17.38 v53.25,18.25
  Top 0.203: R56.1 107.86,5.12 107.57,4.83 105.79,4.83 105.79,7.49 105.56,7.47 R37.R1_2 | U12.8 105.75,12.99 105.79,12.95 v104.9,12.95 | 112.65,11.81 U21.18 | R38.1 117.86,7.87 117.86,7.37 117.6,7.11 116.2,7.11 115.95,7.37 115.95,10.67 115.32,11.3 115.32,12.19 | R26.1 15.96,22.01 | 17.23,21.91 17.14,22 15.98,22 15.96,22.01 | 15.96,22.01 15.95,22.02 16.48,22.02 16.5,22 v16.5,21.25
  Top 0.305: U12.8 106.05,12.95 106.05,11.94 106.02,11.92 105.72,11.92 C26.1 R37.R4_2 | v33,20.5 16.75,20.5 16.5,20.75 v16.5,21.25
  Top 0.406: R37.R1_2 R37.R2_2 R37.R3_2 R37.R4_2 | 112.65,11.81 113.03,12.19 115.32,12.19 115.32,12.95 v115.57,13.21 | R26.1 R27.2 | v102.75,20.12 102.62,20 84.38,20 83.75,19.38 82.38,19.38 82.12,19.62 70.38,19.62 69.12,20.88 64.88,20.88 64.5,20.5 v64.5,19
  Route2 0.165: v55.25,19.25 55,19.25 54.75,19.5 54.75,21 55,21.25 v55.25,21.25
  Route2 0.406: v64.5,19 64,18.5 56,18.5 v55.25,19.25
  Route15 0.305: v46.5,19.62 45.5,20.62 33.12,20.62 v33,20.5
  Route15 0.406: v115.57,13.21 115.57,12.7 115.06,12.19 114.17,12.19 113.92,11.94 105.92,11.94 v104.9,12.95 104.94,12.99
  Bottom 0.203: R100.1 R99.1 114.9,16.6 114.81,16.51 114.81,14.99 | v115.57,13.21 115.57,14.61 115.19,14.99 114.81,14.99 | R98.1 113.41,14.99 114.81,14.99 | v16.5,21.25 16.5,21.88 17.38,22.75 17.38,24.25 17.12,24.5 16.38,24.5 16.25,24.62 U24.5
  Bottom 0.25: C88.2 57.62,18.12 | 57.62,18.25 57.62,18.12 | 57.62,18.12 56.38,18.12 v55.25,19.25
  Bottom 0.305: U24.5 16.26,26.92 15.75,27.43 15.32,27.43 15.25,27.5 15.25,28.16 C66.1 15.4,28.1 | v53.25,18.25 53.25,17.12 52.88,16.75 50.88,16.75 50.5,17.12 50.5,18.25 50.25,18.5 46.88,18.5 46.5,18.88 v46.5,19.62 | v33,20.5 33.24,20.74 34.12,20.74 R136.R1_1 R136.R2_1 R136.R3_1 R136.R4_1 R137.R4_2 R137.R3_2 R137.R2_2 R137.R1_2
  Bottom 0.406: v104.9,12.95 104.9,13.84 103.89,14.86 103.89,16.64 102.75,17.77 v102.75,20.12
+12V
  Route15 1.016: JP2.14 JP2.13
  pour Top (no thermals): 109.86,30.3 109.86,32.77 118.87,32.77 119.89,33.78 122.3,33.78 123.57,32.64 123.57,28.7 114.81,28.7 114.81,29.59 114.05,30.35 111.76,30.35
  pour Bottom (no thermals): 116.84,26.42 116.84,36.45 117.47,37.08 117.47,41.78 117.86,42.16 119.63,42.16 120.02,41.78 120.02,34.29 120.4,33.91 122.3,33.91 123.44,32.89 123.44,30.1 121.79,28.45 121.79,21.08 119.25,18.54 119.25,3.81 118.75,3.3 116.84,3.3 116.84,23.88 118.87,23.88 118.87,26.42
A0_MUX  (via drill 0.25)
  Top 0.203: U21.3 109.6,8.76 109.17,8.38 109.02,8.38 v109.02,8.46 109.02,8.41 108.99,8.38 108.56,8.38 | 108.56,8.38 R37.R2_1 108.31,8.36 108.33,8.38 108.56,8.38
  Bottom 0.203: v109.02,8.46 109.02,8.41 108.99,8.38 108.2,8.38 107.7,7.87 JP3.6
A1_MUX  (via drill 0.25)
  Top 0.203: U21.2 110.39,9.27 109.65,9.27 109.51,9.16 R37.R3_1 107.84,9.16 107.82,9.14 109.02,9.14 | 109.02,9.14 109.12,9.16 | 109.02,9.14 v109.02,9.45 109.02,9.27
  Bottom 0.203: v109.02,9.45 108.13,9.45 107.82,9.14 JP3.7
A2_MUX  (via drill 0.25)
  Top 0.203: 109.02,10.16 110.11,10.16 110.11,9.78 110.36,9.78 U21.1 | R37.R4_1 108.16,10.12 108.2,10.16 109.02,10.16 | 109.02,10.16 v109.02,10.54
  Bottom 0.203: v109.02,10.54 106.93,10.54 JP3.8
ALERTB  (via drill 0.25)
  Top 0.165: U10.L5 53.25,25.25 51.38,25.25 51.25,25.38 50.75,25.38 50.62,25.25 v49.88,25.25 44.12,25.25 42.38,27 37.25,27 | U10.L11 53.25,19.25 52.12,19.25 51.25,20.12 50.25,20.12 50,19.88 v50,19.5 | 37.25,27 36,27 35.62,26.62 21.12,26.62 v21,26.75 | 9.25,19.58 TP19.TP | v37.25,27.25 37.25,27
  Top 0.305: v13.12,24 10.12,24 9.25,23.12 9.25,19.58
  Route2 0.165: v65.75,18.25 65.25,18.25 64.62,17.62 55.62,17.62 54.5,18.75 50.38,18.75 50,19.12 v50,19.5
  Route15 0.165: v65.75,18.25 66.25,18.75 81.62,18.75 82,18.38 84.12,18.38 84.5,18.75 103.75,18.75 105.12,17.38 105.5,17.38 105.52,17.4 v105.54,17.4
  Bottom 0.165: v49.88,25.25 50.12,25 50.12,23.12 50,23 v50,19.5 | U24.1 16.91,22.91 16.62,22.62 10,22.62 9.25,21.88 9.25,19.58 TP19.TP | v21,26.75 20.62,26.75 20.38,27 20.38,28.5 20.12,28.75 19.12,28.75 18,29.88 13.25,29.88 12.75,29.38 12.75,24 v13.12,24 | R137.R4_1 37.58,24.7 37.75,24.88 37.75,27 37.5,27.25 v37.25,27.25
  Bottom 0.203: 105.92,17.4 105.92,14.99 106.43,14.48 106.43,12.19 107.31,11.3 109.47,11.3 109.98,10.79 109.98,8.26 108.33,6.6 108.33,3.72 JP2.3 | JP1.3 108.31,39.13 108.2,39.12 108.2,38.1 106.81,38.1 105.28,36.58 105.28,33.78 105.03,33.53 105.03,20.57 105.92,19.68 105.92,17.4 | v105.54,17.4 105.92,17.4
CTRL  (via drill 0.25)
  Top 0.165: 54.25,17.75 U10.K12 | U10.L12 54.25,17.75 | 54.25,17.75 v54.25,18.25 | v53.25,23.25 U10.L6 | U10.L6 U10.K6 | U10.L6 53.25,24.25 52.38,24.25 52.25,24.38 44,24.38 42.38,26 v38.88,26
  Top 0.203: C36.1 116.97,10.03 117.35,10.41 118.75,10.41 119,10.67 S1.5
  Top 0.406: S1.5 S1.2
  Route15 0.165: v53.25,23.25 53.25,25.62 53.88,26.25 60.5,26.25 62,24.75 62.62,24.75 62.88,25 73.5,25 74,25.5 88.12,25.5 89.25,24.38 89.25,22 89.5,21.75 90,21.75 90.5,22.25 90.5,22.62 90.75,22.88 v103.38,22.88
  Route15 0.203: v104.78,18.54 105.92,18.54 107.44,17.02 107.44,16 108.71,14.73 113.16,14.73 113.67,15.24 114.94,15.24 116.59,13.59 117.22,13.59 118.87,11.94 S1.5
  Bottom 0.165: v54.25,18.25 53.75,18.75 52.12,18.75 51.88,19 51.88,20.38 52.5,21 52.5,22.62 53.12,23.25 v53.25,23.25 | v103.38,22.88 104.27,22.88 | 104.39,18.67 104.39,18.54 v104.78,18.54 | R136.R2_2 37.48,21.6 38.5,22.62 38.5,25.62 v38.88,26
  Bottom 0.203: 105.16,41.15 105.16,37.72 104.52,37.08 104.52,34.29 104.27,34.04 104.27,22.88 104.27,18.8 104.39,18.67 104.39,15.24 105.66,13.97 105.66,12.45 105.28,12.06 105.28,4.95 105.16,4.83 105.16,1.91 105.41,1.65 106.27,1.65 JP2.2 | 105.16,41.15 106.27,41.15 JP1.2 | R135.2 105.16,43.56 105.16,41.15
CTRL_P
  Bottom 0.203: R135.1 107.4,43.22 107.44,43.18 112.27,43.18 113.26,42.19 113.26,38.38 114.55,37.08 TP12.TP
DACP_CH0  (via drill 0.25)
  Top 0.165: v21.75,31 27.38,31 27.88,30.5 28.5,30.5 28.75,30.75 38.62,30.75 39.38,30 39.75,30 40.12,30.38 49.5,30.38 49.88,30 49.88,29.62 v49.88,27.5 | v59.25,23.25 U10.F6
  Route2 0.165: v49.88,27.5 49.88,27.25 50.12,27 52.5,27 52.75,26.75 52.75,26 53,25.75 56.62,25.75 56.75,25.62 56.75,24 57.5,23.25 v59.25,23.25
  Bottom 0.165: VSNSN47.1 21.74,32.26 21.75,32.25 v21.75,31
  Bottom 0.203: R117.2 21.97,33.91 21.72,33.91
  Bottom 0.406: VSNSN47.1 21.72,33.91
DACP_CH1  (via drill 0.25)
  Top 0.165: U10.E6 v60.25,23.25
  Bottom 0.165: v60.25,23.25 60.25,24 59.5,24.75 58.62,24.75 58.25,25.12 58.25,27 57.5,27.75 56.25,27.75 55.75,27.25 55,27.25 54.5,27.75 51.12,27.75 50.12,28.75 50.12,31 49.88,31.25 40.38,31.25 40.12,31 40.12,30.25 39.88,30 39.38,30 39.12,30.25 39.12,31.5 38.88,31.75 33.78,31.75 VSNSN45.1
  Bottom 0.203: R115.2 33.53,33.91 33.27,33.91
  Bottom 0.406: VSNSN45.1 33.27,33.91
DACP_CH2  (via drill 0.25)
  Top 0.165: U10.C6 v61.25,23.25
  Bottom 0.165: v61.25,23.25 60.75,23.75 60.75,24 59.62,25.12 58.88,25.12 58.62,25.38 58.62,27.12 57.62,28.12 56.12,28.12 55.62,27.62 55.12,27.62 54.62,28.12 51.38,28.12 50.5,29 50.5,31.25 50.12,31.62 45,31.62 44.88,31.75 44.88,32.21 VSNSN43.1
  Bottom 0.203: R113.2 45.09,33.91 44.83,33.91
  Bottom 0.406: VSNSN43.1 44.83,33.91
DACP_CH3  (via drill 0.25)
  Top 0.165: U10.D5 v60.25,25.25
  Bottom 0.165: v60.25,25.25 61.5,25.25 62,24.75 62.5,24.75 63.12,25.38 63.12,28.25 62.5,28.88 59.38,28.88 58.5,29.75 57.25,29.75 56.38,30.62 56.38,32.24 VSNSN41.1
  Bottom 0.203: R111.2 56.64,33.91 56.39,33.91
  Bottom 0.406: VSNSN41.1 56.39,33.91
DACP_CH4  (via drill 0.25)
  Top 0.165: U10.E4 60.25,26.25 v62.25,26.25
  Route15 0.165: v62.25,26.25 66.12,26.25 66.75,26.88 67.62,26.88 67.88,26.62 v67.88,26.25
  Bottom 0.165: v67.88,26.25 67.88,32.19 VSNSN39.1
  Bottom 0.203: R109.2 68.2,33.91 67.94,33.91
  Bottom 0.406: VSNSN39.1 67.94,33.91
DACP_CH5  (via drill 0.25)
  Top 0.165: U10.A3 64.38,27.38 79.25,27.38 79.5,27.12 v79.5,26.88
  Bottom 0.165: v79.5,26.88 VSNSN37.1
  Bottom 0.203: R107.2 79.76,33.91 79.5,33.91
  Bottom 0.406: VSNSN37.1 79.5,33.91
DACP_CH6  (via drill 0.25)
  Top 0.165: U10.D3 v61.25,27.25
  Route15 0.165: v61.25,27.25 61.75,26.75 66.12,26.75 66.62,27.25 79.12,27.25 79.25,27.38 91,27.38 v91,27.12
  Bottom 0.165: v91,27.12 91,32.2 VSNSN35.1
  Bottom 0.203: R105.2 91.31,33.91 91.06,33.91
  Bottom 0.406: VSNSN35.1 91.06,33.91
DACP_CH7  (via drill 0.25)
  Top 0.165: U10.E3 60.25,27.25 v60.25,30.5
  Route15 0.165: v60.25,30.5 60.25,31 60.38,31.12 70,31.12 70.38,31.5 101.86,31.5 VSNSN33.1
  Bottom 0.203: R103.2 102.87,33.91 102.62,33.91
  Bottom 0.406: VSNSN33.1 102.62,33.91
DACP_CH8  (via drill 0.25)
  Top 0.165: U10.F12 58.75,17.25 v58.62,17.12
  Route15 0.165: v58.62,17.12 58.62,17.38 58.5,17.5 56.38,17.5 56.12,17.25 56.12,17 55.88,16.75 49.12,16.75 48.75,17.12 47.38,17.12 46.62,16.38 39.38,16.38 39,16.75 38.5,16.75 37.75,16 27.88,16 27.25,16.62 v14.12,16.62
  Bottom 0.165: v14.12,16.62 14.12,14.12 VSNSN32.1
  Bottom 0.203: R97.2 13.21,12.45 13.46,12.45
  Bottom 0.406: 13.46,12.45 13.46,13.72 13.84,14.1 VSNSN32.1
DACP_CH9  (via drill 0.25)
  Top 0.165: U10.E12 59.75,17.12 59.62,17 59.62,15.75 v59.88,15.5
  Route15 0.165: v59.88,15.5 59.62,15.25 25.5,15.25 25.02,14.77 VSNSN30.1
  Bottom 0.203: R95.2 24.77,12.45 25.02,12.45
  Bottom 0.406: 25.02,12.45 VSNSN30.1
DACP_CH10  (via drill 0.25)
  Top 0.165: U10.C12 61.75,15.38 61.25,14.88 v60.75,14.88
  Route15 0.165: v60.75,14.88 60.75,13.62 60.5,13.38 58.38,13.38 58.12,13.62 58.12,14.38 57.62,14.88 36.75,14.88 36.58,14.7 VSNSN28.1
  Bottom 0.203: R93.2 36.32,12.45 36.58,12.45
  Bottom 0.406: 36.58,12.45 VSNSN28.1
DACP_CH11  (via drill 0.25)
  Top 0.165: U10.D11 61.25,18.25 61.25,16.38 v60.75,15.88
  Route15 0.165: v60.75,15.88 60.38,15.88 60.25,16 59.62,16 59.25,15.62 48.12,15.62 v48.12,15.88
  Bottom 0.165: v48.12,15.88 VSNSN26.1
  Bottom 0.203: R91.2 47.88,12.45 48.13,12.45
  Bottom 0.406: 48.13,12.45 VSNSN26.1
DACP_CH12
  Top 0.165: U10.E10 59.25,19.25 59.25,14.54 VSNSN24.1
  Bottom 0.203: R89.2 59.44,12.45 59.69,12.45
  Bottom 0.406: 59.69,12.45 VSNSN24.1
DACP_CH13  (via drill 0.25)
  Top 0.165: U10.A9 64.38,21.38 69.62,21.38 69.88,21.12 v71.12,21.12
  Bottom 0.165: v71.12,21.12 71.12,20.75 71.25,20.62 VSNSN22.1
  Bottom 0.203: R87.2 70.99,12.45 71.25,12.45
  Bottom 0.406: 71.25,12.45 VSNSN22.1
DACP_CH14  (via drill 0.25)
  Top 0.165: U10.D9 v60.25,20.25
  Route15 0.165: v60.25,20.25 82.38,20.25 v82.62,20
  Bottom 0.165: v82.62,20 82.88,19.75 82.88,14.12 82.75,14.15 VSNSN20.1
  Bottom 0.203: R85.2 82.55,12.45 82.8,12.45
  Bottom 0.406: VSNSN20.1 82.8,12.45
DACP_CH15  (via drill 0.25)
  Top 0.165: U10.E9 v59.25,20.25
  Route15 0.165: v59.25,20.25 59.75,19.75 60.88,19.75 61,19.88 82,19.88 82.38,19.5 83.75,19.5 84.12,19.88 93.88,19.88 94.25,19.88 94.5,20.12 v94.5,20.62
  Bottom 0.165: v94.5,20.62 94.38,20.5 94.38,14.11 VSNSN18.1
  Bottom 0.203: R83.2 94.11,12.45 94.36,12.45
  Bottom 0.406: VSNSN18.1 94.36,12.45
EESCL
  Top 0.203: 123.7,6.1 123.44,6.35 R47.1 124.26,6.35 | U22.1 124.04,1.59 124.26,1.78 124.26,6.35 | 124.26,6.35 124.26,6.66 124.84,7.24 124.84,8 125.09,8.26 129.89,8.26 130.4,8.76 130.4,10.29 129.95,10.73 128.24,10.73 J2.11 127.32,9.65
EESDA
  Top 0.203: 123.44,3.43 U22.3 123.38,3.49 123.38,4.76 123.44,4.83 R57.1 122.56,4.83 122.56,7.06 122.68,7.19 124.18,7.19 124.33,7.34 124.33,8.26 124.71,8.64 129.13,8.64 129.41,8.89 129.41,9.65 J2.12
EEVCC  (via drill 0.25)
  Top 0.203: 125.04,20.77 124.43,20.77 C24.1
  Top 0.254: U11.8 U11.7
  Top 0.406: R57.2 R47.2 121.67,6.35 | U22.4 120.58,3.49 120.9,3.56 | 120.9,4.79 R57.2 | 120.9,3.56 120.78,3.56 | 120.9,4.79 120.9,4.83 | 120.9,3.56 120.9,4.79 | R57.2 120.9,4.83 | 120.9,4.83 v120.52,4.83 | 121.67,6.35 121.58,6.35 | 121.67,6.35 121.67,7.87 C35.1
  Top 0.813: 130.14,37.97 130.25,37.95 130.2,37.82 130.3,37.85 130.3,22.61 130.18,22.48 130.12,22.42
  Top 1.016: 130.14,37.97 129.25,38.86 125.86,38.86 125.09,39.62 121.03,39.62 119.76,40.89 119.76,42.55 119.38,42.93 112.78,42.93 112.25,42.4 112.25,41.15 JP1.8 | 130.18,22.48 125.86,22.48 v125.73,22.99 v125.73,21.84 125.86,21.59 125.04,20.77 U11.8
  Route15 0.406: v114.3,19.56 115.82,19.56 118.11,21.84 v125.73,21.84
  Bottom 0.406: D1.2 115.2,19.8 114.81,19.56 v114.3,19.56
  Bottom 0.813: J2.1 127.24,19.7 127.22,19.68 125.83,19.68 arc60 125.73,19.68 v125.73,21.84 v125.73,22.99
  pour Bottom (no thermals): 111.51,2.92 119,2.92 119.76,3.68 119.76,18.29 122.3,20.83 128.11,20.83 128.11,18.92 123.95,18.92 121.54,16.51 121.54,0.76 111.51,0.76
  pour Top (no thermals): 121.92,21.46 124.84,21.46 125.22,21.84 125.22,23.5 126.62,23.5 126.62,21.72 125.09,20.19 121.92,20.19
FAULT  (via drill 0.25)
  Top 0.203: 41.02,18.92 41.06,18.92 R31.2
  Top 0.254: 39.62,18.92 SW2.SW1 | 39.62,18.92 41.02,18.92 41.02,19.81 R29.2 | v39.62,19.68 39.62,18.92
  Bottom 0.254: v39.62,19.68 39.75,19.56 39.75,16.18 Q9.1
FAULTB  (via drill 0.25)
  Top 0.165: U10.M3 U10.M4 | U10.K4 U10.L4 U10.M4 | 54.25,19.75 U10.L10 U10.M10 U10.M9 v50.5,20.75 | v50.5,25.88 50.5,25.75 | 50.5,25.75 U10.M4 | U10.K10 54.25,19.75 | 54.25,19.75 v54.25,20.25 | 50.5,25.75 44.12,25.75 42.5,27.38 38.38,27.38 38,27.75 36.12,27.75 | v21,27.62 21,27.5 21.5,27 35.38,27 36.12,27.75 | v36.12,28.12 36.12,27.75
  Route15 0.165: v54.25,20.25 U10.K10 58.62,19.75 58.75,19.62 58.75,18.88 58.88,18.75 60.62,18.75 61.38,19.5 81.88,19.5 82.25,19.12 83.88,19.12 84.25,19.5 104.75,19.5 104.88,19.62 v104.9,19.68
  Bottom 0.165: v50.5,20.75 50.5,22 51,22.5 51,23 50.5,23.5 v50.5,25.88 | v21,27.62 21,28.88 20.75,29.12 19.38,29.12 18.25,30.25 13,30.25 12.38,29.62 12.38,23.38 | R137.R1_1 36.1,28.1 v36.12,28.12
  Bottom 0.203: JP2.1 106.01,3.72 105.92,3.81 105.92,6.35 105.79,6.48 105.79,11.94 106.05,12.19 106.05,14.22 104.78,15.49 104.78,17.65 105.54,18.41 105.54,19.43 105.28,19.68 v104.9,19.68 104.65,19.68 104.65,33.78 104.9,34.04 104.9,36.83 106.3,38.23 106.3,39.13 JP1.1 | TP21.TP 7.2,12.19 6.89,12.5 6.89,21.75 8.51,23.38 12.38,23.38 15.57,23.38 U24.3
FB_LTC3604
  Top 0.203: 113.45,23.75 R25.2 113.58,24.42 113.79,24.64 114.43,24.64 114.68,24.89 114.68,27.05 114.43,27.3 114.43,28.96 114.03,29.44 U9.11
  Top 0.305: R28.1 C23.1 113.45,23.75 | R25.2 C20.2
GND  (via drill 0.25)
  Top 0.165: v60.25,19.25 U10.D10 U10.C10 | v56.25,21.25 56.25,20.75 | U10.C9 U10.D8 | U10.D6 v61.25,24.25 U10.C5 U10.B6 | v56.25,22.25 56.25,23.75 U10.G6 | U10.D2 61.25,28.25 v61.25,29.5 | v62.25,27.25 62.25,26.75 U10.C3
  Top 0.203: v21.59,13.72 v22.61,13.72 | C27.2 v21.59,13.72 | v21.59,13.72 v20.57,13.72 | v21.59,13.72 21.59,12.2 | R48.1 14.44,6.39 14.35,6.1 | v33.15,13.72 v34.16,13.72 | C28.2 v33.15,13.72 | v33.15,13.72 v32.13,13.72 | v33.15,13.72 33.15,12.2 | R49.1 26,6.39 25.91,6.1 | v44.7,13.72 v45.72,13.72 | C29.2 v44.7,13.72 | v44.7,13.72 v43.69,13.72 | v44.7,13.72 44.7,12.2 | R50.1 37.55,6.39 37.47,6.1 | v56.26,13.72 v57.28,13.72 | C30.2 v56.26,13.72 | v56.26,13.72 v55.24,13.72 | v56.26,13.72 56.26,12.2 | R51.1 49.11,6.39 49.02,6.1 | v67.82,13.72 v68.83,13.72 | C31.2 v67.82,13.72 | v67.82,13.72 v66.8,13.72 | v67.82,13.72 67.82,12.2 | R52.1 60.67,6.39 60.58,6.1 | v79.38,13.72 v80.39,13.72 | C32.2 v79.38,13.72 | v79.38,13.72 v78.36,13.72 | v79.38,13.72 79.38,12.2 | R53.1 72.22,6.39 72.14,6.1 | v90.93,13.72 v91.95,13.72 | C33.2 v90.93,13.72 | v90.93,13.72 v89.92,13.72 | v90.93,13.72 90.93,12.2 | R54.1 83.78,6.39 83.69,6.1 | v102.49,13.72 v103.5,13.72 | C34.2 v102.49,13.72 | v102.49,13.72 v101.47,13.72 | v102.49,13.72 102.49,12.2 | R55.1 95.34,6.39 95.25,6.1 | LED3.N 107.94,19.55 LED3.N 108.58,19.56 108.84,19.81 v108.84,20.07 | v12.57,32.64 v13.59,32.64 | v13.59,32.64 C9.2 | v13.59,32.64 v14.61,32.64 | v13.59,32.64 13.59,34.16 | R9.1 20.74,39.97 20.83,40.26 | v24.13,32.64 v25.15,32.64 | v25.15,32.64 C10.2 | v25.15,32.64 v26.16,32.64 | v25.15,32.64 25.15,34.16 | R10.1 32.3,39.97 32.38,40.26 | v35.69,32.64 v36.7,32.64 | v36.7,32.64 C11.2 | v36.7,32.64 v37.72,32.64 | v36.7,32.64 36.7,34.16 | R11.1 43.85,39.97 43.94,40.26 | v47.24,32.64 v48.26,32.64 | v48.26,32.64 C12.2 | v48.26,32.64 v49.28,32.64 | v48.26,32.64 48.26,34.16 | R12.1 55.41,39.97 55.5,40.26 | v58.8,32.64 v59.82,32.64 | v59.82,32.64 C13.2
  Top 0.203: v59.82,32.64 v60.83,32.64 | v59.82,32.64 59.82,34.16 | R13.1 66.97,39.97 67.06,40.26 | v70.36,32.64 v71.37,32.64 | v71.37,32.64 C14.2 | v71.37,32.64 v72.39,32.64 | v71.37,32.64 71.37,34.16 | R14.1 78.53,39.97 78.61,40.26 | v81.92,32.64 v82.93,32.64 | v82.93,32.64 C15.2 | v82.93,32.64 v83.95,32.64 | v82.93,32.64 82.93,34.16 | R15.1 90.08,39.97 90.17,40.26 | v93.47,32.64 v94.49,32.64 | v94.49,32.64 C16.2 | v94.49,32.64 v95.5,32.64 | v94.49,32.64 94.49,34.16 | R16.1 101.64,39.97 101.73,40.26 | v57.25,27.25 57.25,26.75 U10.H3 | U10.K5 v54.25,25.25 | U10.A10 U10.B9
  Top 0.406: 14.35,6.1 14.48,6.22 14.73,6.22 | v15.49,6.22 14.44,6.22 R48.1 | 25.91,6.1 26.04,6.22 26.29,6.22 | v27.05,6.22 26,6.22 R49.1 | 37.47,6.1 37.59,6.22 37.85,6.22 | v38.61,6.22 37.55,6.22 R50.1 | 49.02,6.1 49.15,6.22 49.4,6.22 | v50.16,6.22 49.11,6.22 R51.1 | 60.58,6.1 60.71,6.22 60.96,6.22 | v61.72,6.22 60.67,6.22 R52.1 | 72.14,6.1 72.26,6.22 72.52,6.22 | v73.28,6.22 72.22,6.22 R53.1 | 83.69,6.1 83.82,6.22 84.07,6.22 | v84.84,6.22 83.78,6.22 R54.1 | 95.25,6.1 95.38,6.22 95.63,6.22 | v96.39,6.22 95.34,6.22 R55.1 | 20.83,40.26 20.7,40.13 20.45,40.13 | v19.68,40.13 20.74,40.13 R9.1 | 32.38,40.26 32.26,40.13 32,40.13 | v31.24,40.13 32.3,40.13 R10.1 | 43.94,40.26 43.81,40.13 43.56,40.13 | v42.8,40.13 43.85,40.13 R11.1 | 55.5,40.26 55.37,40.13 55.12,40.13 | v54.36,40.13 55.41,40.13 R12.1 | 67.06,40.26 66.93,40.13 66.67,40.13 | v65.91,40.13 66.97,40.13 R13.1 | 78.61,40.26 78.49,40.13 78.23,40.13 | v77.47,40.13 78.53,40.13 R14.1 | 90.17,40.26 90.04,40.13 89.79,40.13 | v89.03,40.13 90.08,40.13 R15.1 | 101.73,40.26 101.6,40.13 101.35,40.13 | v100.58,40.13 101.64,40.13 R16.1
  Top 0.813: v66.8,13.72 67.06,13.72
  Bottom 0.203: 22.99,3.03 Q8.2 | 22.99,3.03 22.99,3.05 | v22.99,2.29 22.99,3.03 | 34.54,3.03 Q7.2 | 34.54,3.03 34.54,3.05 | v34.54,2.29 34.54,3.03 | 46.1,3.03 Q6.2 | 46.1,3.03 46.1,3.05 | v46.1,2.29 46.1,3.03 | 57.66,3.03 Q5.2 | 57.66,3.03 57.66,3.05 | v57.66,2.29 57.66,3.03 | 69.22,3.03 Q4.2 | 69.22,3.03 69.22,3.05 | v69.22,2.29 69.22,3.03 | 80.77,3.03 Q3.2 | 80.77,3.03 80.77,3.05 | v80.77,2.29 80.77,3.03 | 92.33,3.03 Q2.2 | 92.33,3.03 92.33,3.05 | v92.33,2.29 92.33,3.03 | 103.89,3.03 Q1.2 | 103.89,3.03 103.89,3.05 | v103.89,2.29 103.89,3.03 | v108.84,20.07 108.58,19.81 | Q17.2 12.19,43.32 | 12.19,43.32 12.19,43.31 | 12.19,43.32 v12.19,44.07 | Q16.2 23.75,43.32 | 23.75,43.32 23.75,43.31 | 23.75,43.32 v23.75,44.07 | Q15.2 35.31,43.32 | 35.31,43.32 35.31,43.31 | 35.31,43.32 v35.31,44.07 | Q14.2 46.86,43.32 | 46.86,43.32 46.86,43.31 | 46.86,43.32 v46.86,44.07 | Q13.2 58.42,43.32 | 58.42,43.32 58.42,43.31 | 58.42,43.32 v58.42,44.07 | Q12.2 69.98,43.32 | 69.98,43.32 69.98,43.31 | 69.98,43.32 v69.98,44.07 | Q11.2 81.53,43.32 | 81.53,43.32 81.53,43.31 | 81.53,43.32 v81.53,44.07 | Q10.2 93.09,43.32 | 93.09,43.32 93.09,43.31 | 93.09,43.32 v93.09,44.07
  Bottom 0.406: 125.95,7.34 125.95,17.78 127.36,17.78 J2.3
  other vias: 112.65,8.76 109.73,15.49 114.55,14.22 111.51,29.21 125.6,7.49 121.79,2.54 119.51,5.21 106.17,25.02 106.17,26.04 117.47,18.29 124.84,18.03 115.57,25.15 116.71,25.15 117.86,25.15 16.89,18.92 60.75,17 56.75,17 62.75,17.12 49.38,20.75 65.25,22.75 48.5,23.5 64.75,28.75 51.75,28.75 65.38,16.25
  pour Top (no thermals): 19.56,14.35 23.11,14.35 23.11,11.05 18.29,11.05 17.65,11.68 17.65,13.34 18.29,13.34 18.29,11.94 18.54,11.68 19.3,11.68 19.56,11.94
  pour Bottom (no thermals): 19.56,14.35 23.11,14.35 23.11,11.18 19.94,11.18 19.56,11.56
  pour Bottom (no thermals): 11.81,5.08 11.81,9.78 13.97,9.78 14.35,10.16 14.35,11.3 16.26,11.3 16.26,9.78 15.88,9.4 15.88,6.1 14.86,5.08
  pour Top (no thermals): 31.11,14.35 34.67,14.35 34.67,11.05 29.84,11.05 29.21,11.68 29.21,13.34 29.84,13.34 29.84,11.94 30.1,11.68 30.86,11.68 31.11,11.94
  pour Bottom (no thermals): 31.11,14.35 34.67,14.35 34.67,11.18 31.5,11.18 31.11,11.56
  pour Bottom (no thermals): 23.62,5.08 23.62,6.73 24,7.11 24,9.78 25.53,9.78 25.91,10.16 25.91,11.3 27.81,11.3 27.81,9.78 27.43,9.4 27.43,6.1 26.42,5.08
  pour Top (no thermals): 42.67,14.35 46.23,14.35 46.23,11.05 41.4,11.05 40.77,11.68 40.77,13.34 41.4,13.34 41.4,11.94 41.66,11.68 42.42,11.68 42.67,11.94
  pour Bottom (no thermals): 42.67,14.35 46.23,14.35 46.23,11.18 43.05,11.18 42.67,11.56
  pour Bottom (no thermals): 35.18,5.08 35.18,6.73 35.56,7.11 35.56,9.78 37.08,9.78 37.47,10.16 37.47,11.3 39.37,11.3 39.37,9.78 38.99,9.4 38.99,6.1 37.97,5.08
  pour Top (no thermals): 54.23,14.35 57.78,14.35 57.78,11.05 52.96,11.05 52.32,11.68 52.32,13.34 52.96,13.34 52.96,11.94 53.21,11.68 53.98,11.68 54.23,11.94
  pour Bottom (no thermals): 54.23,14.35 57.78,14.35 57.78,11.18 54.61,11.18 54.23,11.56
  pour Bottom (no thermals): 46.74,5.08 46.74,6.73 47.12,7.11 47.12,9.78 48.64,9.78 49.02,10.16 49.02,11.3 50.93,11.3 50.93,9.78 50.55,9.4 50.55,6.1 49.53,5.08
  pour Top (no thermals): 65.79,14.35 69.34,14.35 69.34,11.05 64.52,11.05 63.88,11.68 63.88,13.34 64.52,13.34 64.52,11.94 64.77,11.68 65.53,11.68 65.79,11.94
  pour Bottom (no thermals): 65.79,14.35 69.34,14.35 69.34,11.18 66.17,11.18 65.79,11.56
  pour Bottom (no thermals): 58.29,5.08 58.29,6.73 58.67,7.11 58.67,9.78 60.2,9.78 60.58,10.16 60.58,11.3 62.48,11.3 62.48,9.78 62.1,9.4 62.1,6.1 61.09,5.08
  pour Top (no thermals): 77.34,14.35 80.9,14.35 80.9,11.05 76.07,11.05 75.44,11.68 75.44,13.34 76.07,13.34 76.07,11.94 76.33,11.68 77.09,11.68 77.34,11.94
  pour Bottom (no thermals): 77.34,14.35 80.9,14.35 80.9,11.18 77.72,11.18 77.34,11.56
  pour Bottom (no thermals): 69.85,5.08 69.85,6.73 70.23,7.11 70.23,9.78 71.75,9.78 72.14,10.16 72.14,11.3 74.04,11.3 74.04,9.78 73.66,9.4 73.66,6.1 72.64,5.08
  pour Top (no thermals): 88.9,14.35 92.46,14.35 92.46,11.05 87.63,11.05 87,11.68 87,13.34 87.63,13.34 87.63,11.94 87.88,11.68 88.65,11.68 88.9,11.94
  pour Bottom (no thermals): 88.9,14.35 92.46,14.35 92.46,11.18 89.28,11.18 88.9,11.56
  pour Bottom (no thermals): 81.41,5.08 81.41,6.73 81.79,7.11 81.79,9.78 83.31,9.78 83.69,10.16 83.69,11.3 85.6,11.3 85.6,9.78 85.22,9.4 85.22,6.1 84.2,5.08
  pour Top (no thermals): 100.46,14.35 104.01,14.35 104.01,11.05 99.19,11.05 98.55,11.68 98.55,13.34 99.19,13.34 99.19,11.94 99.44,11.68 100.2,11.68 100.46,11.94
  pour Bottom (no thermals): 100.46,14.35 104.27,14.35 104.27,11.18 100.84,11.18 100.46,11.56
  pour Bottom (no thermals): 92.96,5.08 92.96,6.73 93.34,7.11 93.34,9.78 94.87,9.78 95.25,10.16 95.25,11.3 97.16,11.3 97.16,9.78 96.77,9.4 96.77,6.1 95.76,5.08
  pour Route2 (no thermals): 0.89,45.59 0.89,3.05 3.17,0.76 130.65,0.76 130.65,45.59
  pour Bottom (no thermals): 11.94,32 103.89,32 103.89,41.27 104.27,41.27 104.27,44.58 103.89,44.58 103.89,45.59 130.65,45.59 130.65,0.76 122.05,0.76 122.05,16.38 124.08,18.41 128.49,18.41 128.52,21.34 122.3,21.34 122.3,28.19 123.95,29.84 123.95,33.15 122.56,34.42 120.65,34.42 120.52,34.54 120.52,41.91 119.76,42.67 117.73,42.67 117.09,42.04 117.09,37.34 116.46,36.7 116.46,25.91 118.36,25.91 118.36,24.38 116.46,24.38 116.46,3.3 111.12,3.3 111.12,0.76 104.27,0.76 104.27,14.35 11.81,14.35 11.81,5.08 11.3,5.08 11.3,1.78 11.81,1.78 11.81,0.76 0.89,0.76 0.89,45.59 11.81,45.59 11.81,41.53 11.3,41.53 11.3,35.81 11.94,35.18
  pour Top (no thermals): 104.01,14.35 65.91,14.35 65.91,30.86 50.29,30.86 50.29,14.35 11.81,14.35 11.81,0.76 1.78,0.76 0.89,1.65 0.89,45.59 11.81,45.59 11.81,32 105.16,32 105.16,26.42 106.3,26.42 106.55,26.16 106.55,19.18 127.13,19.18 127.13,27.56 124.08,27.56 124.08,32.77 122.43,34.29 119.63,34.29 118.62,33.27 109.35,33.27 109.35,32.38 105.16,32.38 105.16,32.13 104.01,32.13 104.01,45.59 130.65,45.59 130.65,0.76 104.01,0.76 104.01,6.35 104.52,6.35 104.52,11.05 104.01,11.05
  pour Top (no thermals): 110.74,29.84 113.92,29.84 114.43,29.34 114.43,28.19 124.08,28.19 124.08,27.56 118.24,27.56 118.24,24.26 123.06,24.26 123.83,23.5 124.71,23.5 124.71,21.97 124.59,21.84 111.51,21.84 111.51,25.02 110.74,25.02
  pour Bottom (no thermals): 23.37,41.27 23.37,36.58 21.21,36.58 20.83,36.2 20.83,35.05 18.92,35.05 18.92,36.58 19.3,36.96 19.3,40.26 20.32,41.27
  pour Top (no thermals): 15.62,32 11.94,32 11.94,35.31 16.89,35.31 17.53,34.67 17.53,33.02 16.89,33.02 16.89,34.42 16.64,34.67 15.88,34.67 15.62,34.42
  pour Bottom (no thermals): 15.62,32 12.06,32 12.06,35.18 15.24,35.18 15.62,34.8
  pour Bottom (no thermals): 34.92,41.27 34.92,36.58 32.77,36.58 32.38,36.2 32.38,35.05 30.48,35.05 30.48,36.58 30.86,36.96 30.86,40.26 31.88,41.27
  pour Top (no thermals): 27.18,32 23.62,32 23.62,35.31 28.45,35.31 29.08,34.67 29.08,33.02 28.45,33.02 28.45,34.42 28.19,34.67 27.43,34.67 27.18,34.42
  pour Bottom (no thermals): 27.18,32 23.62,32 23.62,35.18 26.8,35.18 27.18,34.8
  pour Bottom (no thermals): 46.48,41.27 46.48,36.58 44.32,36.58 43.94,36.2 43.94,35.05 42.04,35.05 42.04,36.58 42.42,36.96 42.42,40.26 43.43,41.27
  pour Top (no thermals): 38.73,32 35.18,32 35.18,35.31 40.01,35.31 40.64,34.67 40.64,33.02 40.01,33.02 40.01,34.42 39.75,34.67 38.99,34.67 38.73,34.42
  pour Bottom (no thermals): 38.73,32 35.18,32 35.18,35.18 38.35,35.18 38.73,34.8
  pour Bottom (no thermals): 58.04,41.27 58.04,36.58 55.88,36.58 55.5,36.2 55.5,35.05 53.59,35.05 53.59,36.58 53.98,36.96 53.98,40.26 54.99,41.27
